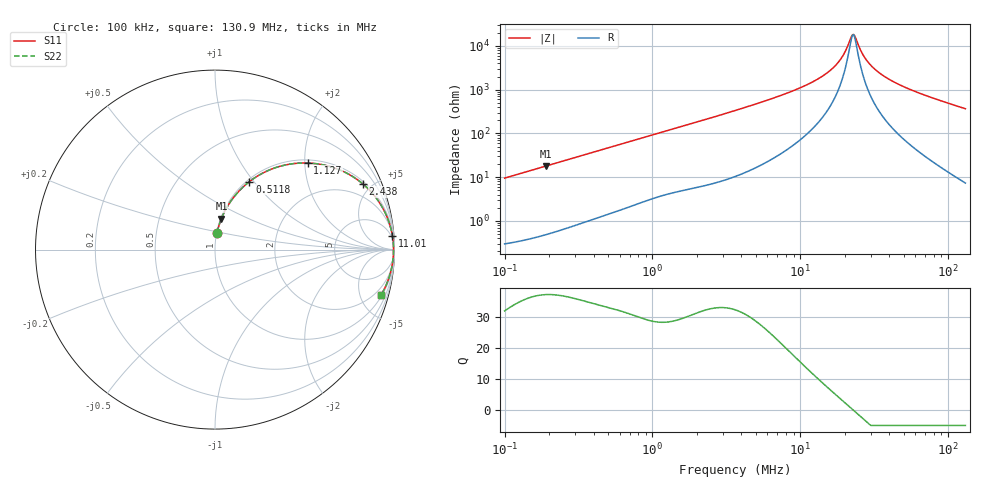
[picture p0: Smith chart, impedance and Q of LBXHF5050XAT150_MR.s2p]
! LBXHF5050XAT150_MR  S-PARAMETER MODEL  ( Standard Model )
! Model Generated by TAIYO YUDEN Corporation (http://www.ty-top.com)
! Version 1.0
! TAIYO YUDEN Control No. 44861
! Copyright(c) 2022 TAIYO YUDEN CO.,LTD. All Rights Reserved.
! Product Description (link to TY-COMPAS)
! https://ds.yuden.co.jp/TYCOMPAS/or/detail?pn=LBXHF5050XAT150MMR&u=M
! Products Name : Inductors
! Characteristics :
!  Inductance : 15 [uH] , SRF(min) : 17 [MHz] , DC Resistance(max) : 0.18 [Ohm]
!  Rated Current : Saturation  2000 [mA] , Temp Rise  860 [mA]
!  Case Size : 5.0 x 5.0 / 0.197 x 0.197 [mm/inch] , Thickness : 3.1 / 0.122 [mm/inch]
!  (Conditions: Temperature = 25 [degC] , DC Bias Current = 0 [A])
! External Node Assignments :
!  1  o---GGG---o  2
! GND o---------o GND
! Frequency Range : 0.1MHz  -  130.914307MHz  [ 402 STEP ]
# MHz S RI R 50
! Freq[MHz].  S11 Real  S11 Imag  S21 Real  S21 Imag  S12 Real  S12 Imag  S22 Real  S22 Imag
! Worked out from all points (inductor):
!   401 points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, 100 kHz to 130.9 MHz, reference 50 ohm
!   read as one part in series: L = 15.1 uH near 103.7 kHz
!   highest Q = 37.2 at 190.8 kHz (marker M1), where L = 15 uH
!   self-resonance near 22.56 MHz
!   S11 on the Smith chart (normalised r, x): 100 kHz: 1.01, +0.19; 511.8 kHz: 1.03, +0.95; 1.127 MHz: 1.07, +2.06; 2.438 MHz: 1.14, +4.43; 11.01 MHz: 3, +26; 130.9 MHz: 1.15, -7.33
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0.1  0.0118 0.0934  0.9882 -0.0934  0.9882 -0.0934  0.0118 0.0934
0.190778  0.0357 0.1726  0.9643 -0.1726  0.9643 -0.1726  0.0357 0.1726
0.332733  0.0951 0.2796  0.9049 -0.2796  0.9049 -0.2796  0.0951 0.2796
0.511817  0.1922 0.3792  0.8078 -0.3792  0.8078 -0.3792  0.1922 0.3792
1.10711  0.507 0.4826  0.493 -0.4826  0.493 -0.4826  0.507 0.4826
1.127154  0.5154 0.4824  0.4846 -0.4824  0.4846 -0.4824  0.5154 0.4824
2.438144  0.8234 0.3663  0.1766 -0.3663  0.1766 -0.3663  0.8234 0.3663
3.683715  0.9129 0.2669  0.0871 -0.2669  0.0871 -0.2669  0.9129 0.2669
11.00592  0.9883 0.0766  0.0117 -0.0766  0.0117 -0.0766  0.9883 0.0766
12.03896  0.99 0.066  0.01 -0.066  0.01 -0.066  0.99 0.066
14.93133  0.9927 0.0423  0.00733 -0.0423  0.00733 -0.0423  0.9927 0.0423
17.54812  0.9939 0.0257  0.00613 -0.0257  0.00613 -0.0257  0.9939 0.0257
19.54274  0.9943 0.0151  0.00566 -0.0151  0.00566 -0.0151  0.9943 0.0151
22.15811  0.9946 0.00282  0.00541 -0.00282  0.00541 -0.00282  0.9946 0.00282
22.96771  0.9946 -0.000657  0.0054 0.000657  0.0054 0.000657  0.9946 -0.000657
23.80689  0.9946 -0.00414  0.00541 0.00414  0.00541 0.00414  0.9946 -0.00414
26.51291  0.9944 -0.0146  0.00559 0.0146  0.00559 0.0146  0.9944 -0.0146
29.00146  0.9941 -0.0235  0.00591 0.0235  0.00591 0.0235  0.9941 -0.0235
33.478  0.9932 -0.0381  0.00681 0.0381  0.00681 0.0381  0.9932 -0.0381
40.05754  0.9913 -0.0573  0.00865 0.0573  0.00865 0.0573  0.9913 -0.0573
65.02508  0.9801 -0.1195  0.0199 0.1195  0.0199 0.1195  0.9801 -0.1195
130.9143  0.9264 -0.2513  0.0736 0.2513  0.0736 0.2513  0.9264 -0.2513
